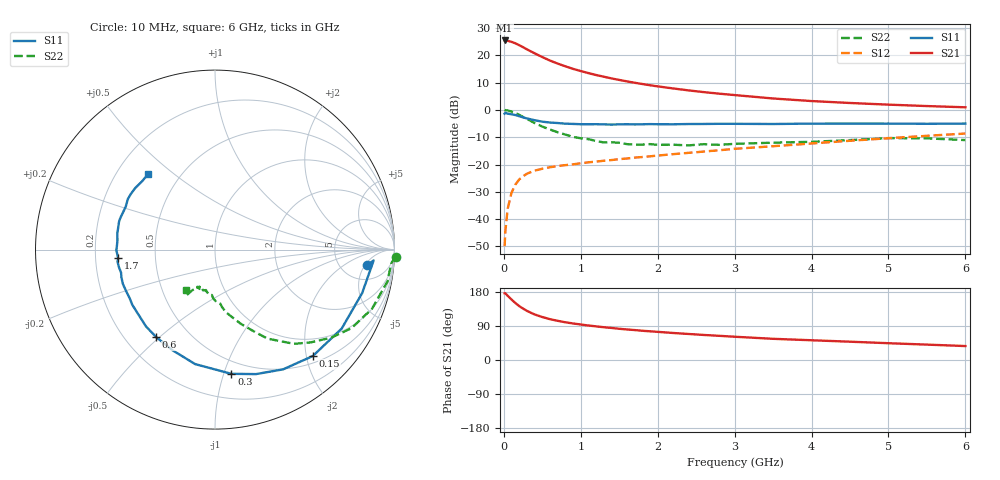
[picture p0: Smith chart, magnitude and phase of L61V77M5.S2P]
!  INFINEON TECHNOLOGIES Small Signal Semiconductors
! BFR380L3 , Si-NPN RF-Transistor in TSLP-3-1
!  Vce=1.75 V,  Ic=7.5 mA
! Common Emitter S-Parameters:  07. March 2005
#  GHz  S  MA  R  50
! f  S11  S21  S12  S22
! GHz  Mag  Ang  Mag  Ang  Mag  Ang  Mag  Ang
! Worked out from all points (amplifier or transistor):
!   36 points, 10 MHz to 6 GHz, reference 50 ohm
!   highest |S21| = 25.4 dB at 10 MHz (marker M1)
!   |S21| within 3 dB of that: start of sweep to 284.1 MHz
!   unconditionally stable (mu >= 1): 2.258 GHz to 4.831 GHz
!   at 250 MHz: K = 0.21, MSG = 23.6 dB, |S12| = -24.3 dB
!   at 1.4 GHz: K = 0.84, MSG = 14.9 dB, |S12| = -18.4 dB
!   at 6 GHz: K = 0.96, MSG = 4.8 dB, |S12| = -8.7 dB
!   S11 on the Smith chart (normalised r, x): 10 MHz: 9, -6; 150 MHz: 0.63, -2.12; 300 MHz: 0.39, -1.06; 600 MHz: 0.33, -0.49; 1.7 GHz: 0.30, -0.04; 6 GHz: 0.33, +0.41
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0.01  0.8526 -5.8  18.69 176.1  0.0032 83.8  1.008 -2.2
0.02  0.8859 -3.9  18.62 176.0  0.0061 87.3  0.9852 -4.4
0.05  0.8549 -16.5  18.4 169.4  0.0155 83.3  0.9769 -10.5
0.1  0.8318 -31.9  17.61 159.6  0.0305 74.3  0.935 -20.6
0.15  0.8054 -47.4  16.58 150.3  0.043 66.9  0.8777 -29.9
0.2  0.7674 -60.4  15.31 142.3  0.0533 62.4  0.8128 -37.1
0.25  0.7302 -71.8  14.08 135.7  0.061 57.2  0.7419 -44.2
0.3  0.698 -82.5  12.86 129.6  0.0679 53.6  0.6853 -50.0
0.4  0.6475 -99.8  10.87 120.2  0.0774 48.4  0.5756 -59.5
0.5  0.6089 -112.8  9.277 113.4  0.0837 45.4  0.4958 -65.3
0.6  0.5874 -123.9  7.999 107.7  0.0892 44.0  0.437 -70.9
0.7  0.5752 -132.0  7.047 103.4  0.0939 43.8  0.3898 -75.6
0.8  0.5596 -139.5  6.281 99.5  0.0975 43.5  0.3536 -80.2
1.1  0.5466 -155.3  4.715 91.0  0.1097 45.0  0.291 -88.7
1.4  0.5388 -166.2  3.769 84.6  0.1207 47.2  0.2552 -95.0
1.7  0.5423 -174.9  3.144 79.0  0.1338 49.4  0.2306 -102.5
2.2  0.546 174.4  2.472 71.3  0.1549 52.8  0.2307 -107.7
2.8  0.5567 164.0  1.983 63.8  0.1825 56.0  0.2293 -115.4
3.5  0.5519 154.3  1.619 55.9  0.2163 57.1  0.2513 -118.0
4.5  0.5622 146.6  1.339 48.3  0.2725 58.9  0.28 -120.8
5.5  0.5567 137.2  1.176 40.6  0.3355 57.6  0.3013 -123.4
6  0.562 131.6  1.117 36.8  0.3694 56.2  0.2802 -125.8
